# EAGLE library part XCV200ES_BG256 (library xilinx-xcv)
xcv200es_bg256 edit this description Auto generated by make-symbol-device-package-bsdl.ulp Rev. 26 Source: xcv200es_bg256.bsd
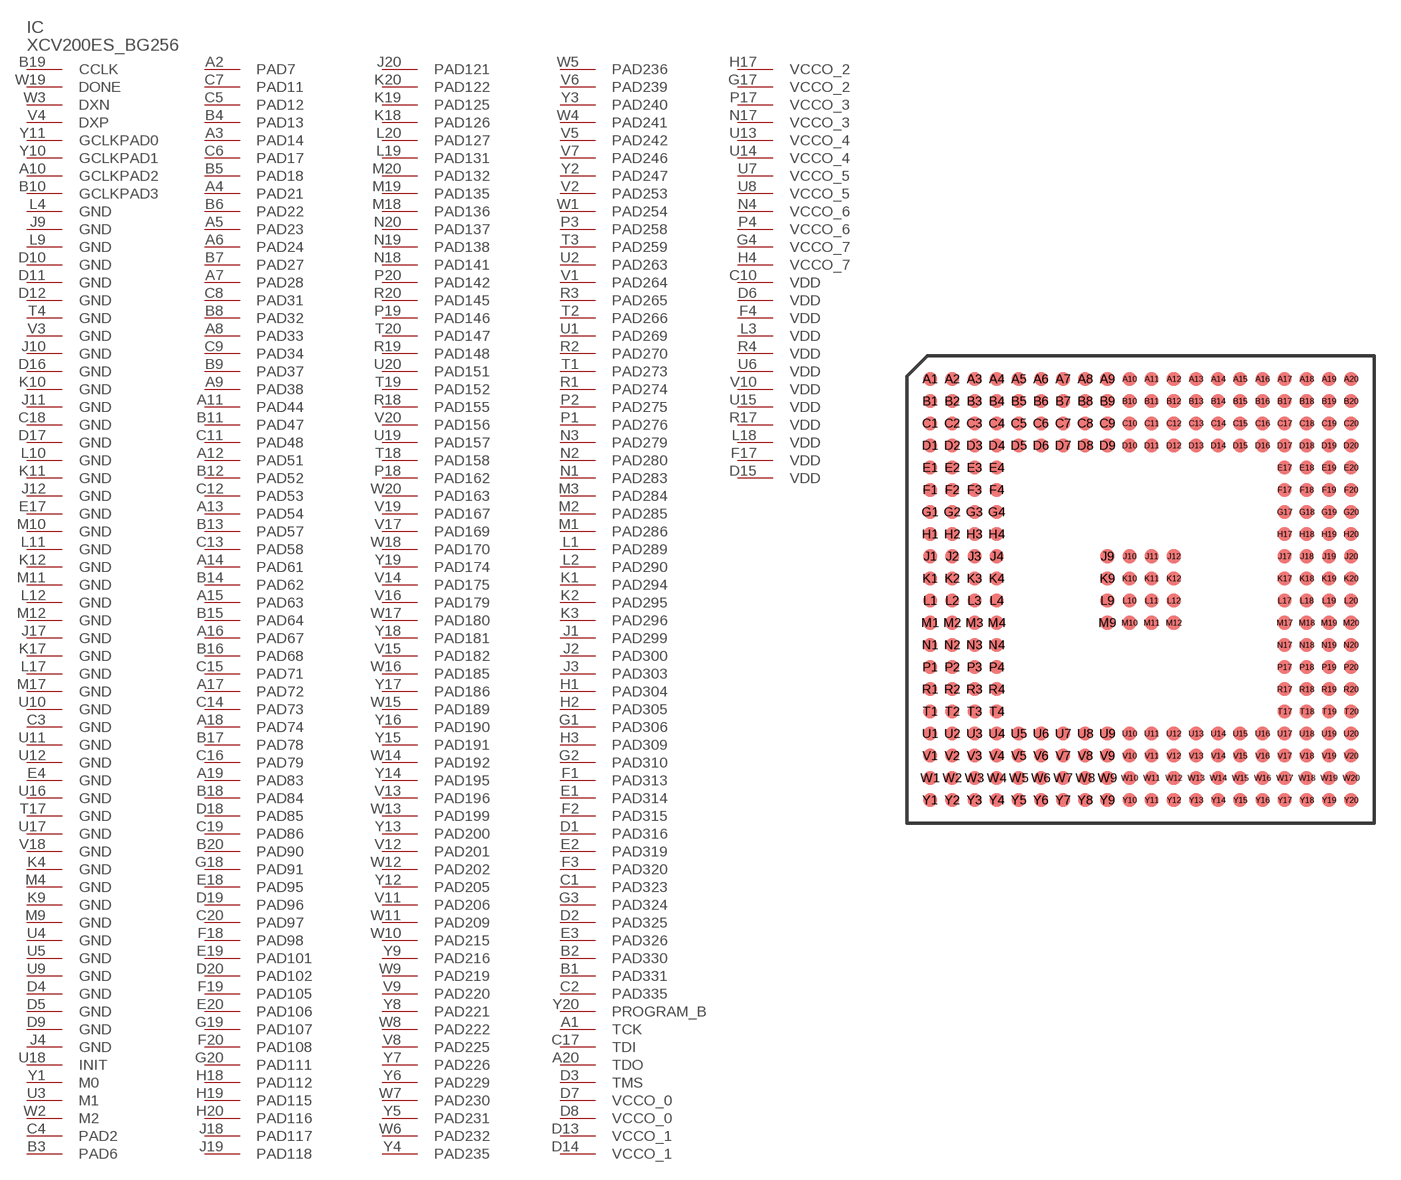
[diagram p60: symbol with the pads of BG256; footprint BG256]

Designator prefix IC

## XCV200ES_BG256 (OC_FARNELL: unknown; OC_NEWARK: unknown)  [BG256]
A1  TCK  in
A2  PAD7
A3  PAD14
A4  PAD21
A5  PAD23
A6  PAD24
A7  PAD28
A8  PAD33
A9  PAD38
A10  GCLKPAD2  in
A11  PAD44
A12  PAD51
A13  PAD54
A14  PAD61
A15  PAD63
A16  PAD67
A17  PAD72
A18  PAD74
A19  PAD83
A20  TDO  out
B1  PAD331
B2  PAD330
B3  PAD6
B4  PAD13
B5  PAD18
B6  PAD22
B7  PAD27
B8  PAD32
B9  PAD37
B10  GCLKPAD3  in
B11  PAD47
B12  PAD52
B13  PAD57
B14  PAD62
B15  PAD64
B16  PAD68
B17  PAD78
B18  PAD84
B19  CCLK
B20  PAD90
C1  PAD323
C2  PAD335
C3  GND  pwr
C4  PAD2
C5  PAD12
C6  PAD17
C7  PAD11
C8  PAD31
C9  PAD34
C10  VDD  pwr
C11  PAD48
C12  PAD53
C13  PAD58
C14  PAD73
C15  PAD71
C16  PAD79
C17  TDI  in
C18  GND  pwr
C19  PAD86
C20  PAD97
D1  PAD316
D2  PAD325
D3  TMS  in
D4  GND  pwr
D5  GND  pwr
D6  VDD  pwr
D7  VCCO_0  pwr
D8  VCCO_0  pwr
D9  GND  pwr
D10  GND  pwr
D11  GND  pwr
D12  GND  pwr
D13  VCCO_1  pwr
D14  VCCO_1  pwr
D15  VDD  pwr
D16  GND  pwr
D17  GND  pwr
D18  PAD85
D19  PAD96
D20  PAD102
E1  PAD314
E2  PAD319
E3  PAD326
E4  GND  pwr
E17  GND  pwr
E18  PAD95
E19  PAD101
E20  PAD106
F1  PAD313
F2  PAD315
F3  PAD320
F4  VDD  pwr
F17  VDD  pwr
F18  PAD98
F19  PAD105
F20  PAD108
G1  PAD306
G2  PAD310
G3  PAD324
G4  VCCO_7  pwr
G17  VCCO_2  pwr
G18  PAD91
G19  PAD107
G20  PAD111
H1  PAD304
H2  PAD305
H3  PAD309
H4  VCCO_7  pwr
H17  VCCO_2  pwr
H18  PAD112
H19  PAD115
H20  PAD116
J1  PAD299
J2  PAD300
J3  PAD303
J4  GND  pwr
J9  GND  pwr
J10  GND  pwr
J11  GND  pwr
J12  GND  pwr
J17  GND  pwr
J18  PAD117
J19  PAD118
J20  PAD121
K1  PAD294
K2  PAD295
K3  PAD296
K4  GND  pwr
K9  GND  pwr
K10  GND  pwr
K11  GND  pwr
K12  GND  pwr
K17  GND  pwr
K18  PAD126
K19  PAD125
K20  PAD122
L1  PAD289
L2  PAD290
L3  VDD  pwr
L4  GND  pwr
L9  GND  pwr
L10  GND  pwr
L11  GND  pwr
L12  GND  pwr
L17  GND  pwr
L18  VDD  pwr
L19  PAD131
L20  PAD127
M1  PAD286
M2  PAD285
M3  PAD284
M4  GND  pwr
M9  GND  pwr
M10  GND  pwr
M11  GND  pwr
M12  GND  pwr
M17  GND  pwr
M18  PAD136
M19  PAD135
M20  PAD132
N1  PAD283
N2  PAD280
N3  PAD279
N4  VCCO_6  pwr
N17  VCCO_3  pwr
N18  PAD141
N19  PAD138
N20  PAD137
P1  PAD276
P2  PAD275
P3  PAD258
P4  VCCO_6  pwr
P17  VCCO_3  pwr
P18  PAD162
P19  PAD146
P20  PAD142
R1  PAD274
R2  PAD270
R3  PAD265
R4  VDD  pwr
R17  VDD  pwr
R18  PAD155
R19  PAD148
R20  PAD145
T1  PAD273
T2  PAD266
T3  PAD259
T4  GND  pwr
T17  GND  pwr
T18  PAD158
T19  PAD152
T20  PAD147
U1  PAD269
U2  PAD263
U3  M1  in
U4  GND  pwr
U5  GND  pwr
U6  VDD  pwr
U7  VCCO_5  pwr
U8  VCCO_5  pwr
U9  GND  pwr
U10  GND  pwr
U11  GND  pwr
U12  GND  pwr
U13  VCCO_4  pwr
U14  VCCO_4  pwr
U15  VDD  pwr
U16  GND  pwr
U17  GND  pwr
U18  INIT
U19  PAD157
U20  PAD151
V1  PAD264
V2  PAD253
V3  GND  pwr
V4  DXP  pas
V5  PAD242
V6  PAD239
V7  PAD246
V8  PAD225
V9  PAD220
V10  VDD  pwr
V11  PAD206
V12  PAD201
V13  PAD196
V14  PAD175
V15  PAD182
V16  PAD179
V17  PAD169
V18  GND  pwr
V19  PAD167
V20  PAD156
W1  PAD254
W2  M2  in
W3  DXN  pas
W4  PAD241
W5  PAD236
W6  PAD232
W7  PAD230
W8  PAD222
W9  PAD219
W10  PAD215
W11  PAD209
W12  PAD202
W13  PAD199
W14  PAD192
W15  PAD189
W16  PAD185
W17  PAD180
W18  PAD170
W19  DONE
W20  PAD163
Y1  M0  in
Y2  PAD247
Y3  PAD240
Y4  PAD235
Y5  PAD231
Y6  PAD229
Y7  PAD226
Y8  PAD221
Y9  PAD216
Y10  GCLKPAD1  in
Y11  GCLKPAD0  in
Y12  PAD205
Y13  PAD200
Y14  PAD195
Y15  PAD191
Y16  PAD190
Y17  PAD186
Y18  PAD181
Y19  PAD174
Y20  PROGRAM_B  in

## Footprint BG256 (pad centres in mm)
xcv100_bg256_1532 edit this description Auto generated by make-symbol-device-package-bsdl.ulp Rev. 25 Source: xcv100_bg256_1532.bsd
smd 0.8 x 0.8: A1 -12.065,12.065; A2 -10.795,12.065; A3 -9.525,12.065; A4 -8.255,12.065; A5 -6.985,12.065; A6 -5.715,12.065; A7 -4.445,12.065; A8 -3.175,12.065; A9 -1.905,12.065; A10 -0.635,12.065; A11 0.635,12.065; A12 1.905,12.065; A13 3.175,12.065; A14 4.445,12.065; A15 5.715,12.065; A16 6.985,12.065; A17 8.255,12.065; A18 9.525,12.065; A19 10.795,12.065; A20 12.065,12.065; B1 -12.065,10.795; B2 -10.795,10.795; B3 -9.525,10.795; B4 -8.255,10.795; B5 -6.985,10.795; B6 -5.715,10.795; B7 -4.445,10.795; B8 -3.175,10.795; B9 -1.905,10.795; B10 -0.635,10.795; B11 0.635,10.795; B12 1.905,10.795; B13 3.175,10.795; B14 4.445,10.795; B15 5.715,10.795; B16 6.985,10.795; B17 8.255,10.795; B18 9.525,10.795; B19 10.795,10.795; B20 12.065,10.795; C1 -12.065,9.525; C2 -10.795,9.525; C3 -9.525,9.525; C4 -8.255,9.525; C5 -6.985,9.525; C6 -5.715,9.525; C7 -4.445,9.525; C8 -3.175,9.525; C9 -1.905,9.525; C10 -0.635,9.525; C11 0.635,9.525; C12 1.905,9.525; C13 3.175,9.525; C14 4.445,9.525; C15 5.715,9.525; C16 6.985,9.525; C17 8.255,9.525; C18 9.525,9.525; C19 10.795,9.525; C20 12.065,9.525; D1 -12.065,8.255; D2 -10.795,8.255; D3 -9.525,8.255; D4 -8.255,8.255; D5 -6.985,8.255; D6 -5.715,8.255; D7 -4.445,8.255; D8 -3.175,8.255; D9 -1.905,8.255; D10 -0.635,8.255; D11 0.635,8.255; D12 1.905,8.255; D13 3.175,8.255; D14 4.445,8.255; D15 5.715,8.255; D16 6.985,8.255; D17 8.255,8.255; D18 9.525,8.255; D19 10.795,8.255; D20 12.065,8.255; E1 -12.065,6.985; E2 -10.795,6.985; E3 -9.525,6.985; E4 -8.255,6.985; E17 8.255,6.985; E18 9.525,6.985; E19 10.795,6.985; E20 12.065,6.985; F1 -12.065,5.715; F2 -10.795,5.715; F3 -9.525,5.715; F4 -8.255,5.715; F17 8.255,5.715; F18 9.525,5.715; F19 10.795,5.715; F20 12.065,5.715; G1 -12.065,4.445; G2 -10.795,4.445; G3 -9.525,4.445; G4 -8.255,4.445; G17 8.255,4.445; G18 9.525,4.445; G19 10.795,4.445; G20 12.065,4.445; H1 -12.065,3.175; H2 -10.795,3.175; H3 -9.525,3.175; H4 -8.255,3.175; H17 8.255,3.175; H18 9.525,3.175; H19 10.795,3.175; H20 12.065,3.175; J1 -12.065,1.905; J2 -10.795,1.905; J3 -9.525,1.905; J4 -8.255,1.905; J9 -1.905,1.905; J10 -0.635,1.905; J11 0.635,1.905; J12 1.905,1.905; J17 8.255,1.905; J18 9.525,1.905; J19 10.795,1.905; J20 12.065,1.905; K1 -12.065,0.635; K2 -10.795,0.635; K3 -9.525,0.635; K4 -8.255,0.635; K9 -1.905,0.635; K10 -0.635,0.635; K11 0.635,0.635; K12 1.905,0.635; K17 8.255,0.635; K18 9.525,0.635; K19 10.795,0.635; K20 12.065,0.635; L1 -12.065,-0.635; L2 -10.795,-0.635; L3 -9.525,-0.635; L4 -8.255,-0.635; L9 -1.905,-0.635; L10 -0.635,-0.635; L11 0.635,-0.635; L12 1.905,-0.635; L17 8.255,-0.635; L18 9.525,-0.635; L19 10.795,-0.635; L20 12.065,-0.635; M1 -12.065,-1.905; M2 -10.795,-1.905; M3 -9.525,-1.905; M4 -8.255,-1.905; M9 -1.905,-1.905; M10 -0.635,-1.905; M11 0.635,-1.905; M12 1.905,-1.905; M17 8.255,-1.905; M18 9.525,-1.905; M19 10.795,-1.905; M20 12.065,-1.905; N1 -12.065,-3.175; N2 -10.795,-3.175; N3 -9.525,-3.175; N4 -8.255,-3.175; N17 8.255,-3.175; N18 9.525,-3.175; N19 10.795,-3.175; N20 12.065,-3.175; P1 -12.065,-4.445; P2 -10.795,-4.445; P3 -9.525,-4.445; P4 -8.255,-4.445; P17 8.255,-4.445; P18 9.525,-4.445; P19 10.795,-4.445; P20 12.065,-4.445; R1 -12.065,-5.715; R2 -10.795,-5.715; R3 -9.525,-5.715; R4 -8.255,-5.715; R17 8.255,-5.715; R18 9.525,-5.715; R19 10.795,-5.715; R20 12.065,-5.715; T1 -12.065,-6.985; T2 -10.795,-6.985; T3 -9.525,-6.985; T4 -8.255,-6.985; T17 8.255,-6.985; T18 9.525,-6.985; T19 10.795,-6.985; T20 12.065,-6.985; U1 -12.065,-8.255; U2 -10.795,-8.255; U3 -9.525,-8.255; U4 -8.255,-8.255; U5 -6.985,-8.255; U6 -5.715,-8.255; U7 -4.445,-8.255; U8 -3.175,-8.255; U9 -1.905,-8.255; U10 -0.635,-8.255; U11 0.635,-8.255; U12 1.905,-8.255; U13 3.175,-8.255; U14 4.445,-8.255; U15 5.715,-8.255; U16 6.985,-8.255; U17 8.255,-8.255; U18 9.525,-8.255; U19 10.795,-8.255; U20 12.065,-8.255; V1 -12.065,-9.525; V2 -10.795,-9.525; V3 -9.525,-9.525; V4 -8.255,-9.525; V5 -6.985,-9.525; V6 -5.715,-9.525; V7 -4.445,-9.525; V8 -3.175,-9.525; V9 -1.905,-9.525; V10 -0.635,-9.525; V11 0.635,-9.525; V12 1.905,-9.525; V13 3.175,-9.525; V14 4.445,-9.525; V15 5.715,-9.525; V16 6.985,-9.525; V17 8.255,-9.525; V18 9.525,-9.525; V19 10.795,-9.525; V20 12.065,-9.525; W1 -12.065,-10.795; W2 -10.795,-10.795; W3 -9.525,-10.795; W4 -8.255,-10.795; W5 -6.985,-10.795; W6 -5.715,-10.795; W7 -4.445,-10.795; W8 -3.175,-10.795; W9 -1.905,-10.795; W10 -0.635,-10.795; W11 0.635,-10.795; W12 1.905,-10.795; W13 3.175,-10.795; W14 4.445,-10.795; W15 5.715,-10.795; W16 6.985,-10.795; W17 8.255,-10.795; W18 9.525,-10.795; W19 10.795,-10.795; W20 12.065,-10.795; Y1 -12.065,-12.065; Y2 -10.795,-12.065; Y3 -9.525,-12.065; Y4 -8.255,-12.065; Y5 -6.985,-12.065; Y6 -5.715,-12.065; Y7 -4.445,-12.065; Y8 -3.175,-12.065; Y9 -1.905,-12.065; Y10 -0.635,-12.065; Y11 0.635,-12.065; Y12 1.905,-12.065; Y13 3.175,-12.065; Y14 4.445,-12.065; Y15 5.715,-12.065; Y16 6.985,-12.065; Y17 8.255,-12.065; Y18 9.525,-12.065; Y19 10.795,-12.065; Y20 12.065,-12.065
